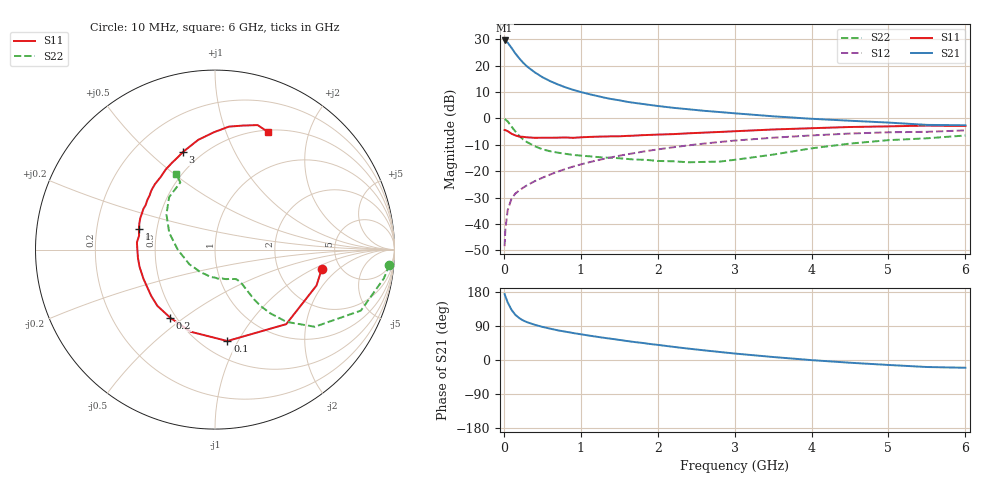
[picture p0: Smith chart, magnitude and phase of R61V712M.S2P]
! SIEMENS Small Signal Semiconductors
! BFR193
! Si NPN RF Bipolar Junction Transistor in SOT23
! VCE = 1.75 V  IC = 12 mA
! Common Emitter S-Parameters:  May  1996
# GHz  S  MA  R  50
!  f  S11  S21  S12  S22
! GHz  MAG  ANG  MAG  ANG  MAG  ANG  MAG  ANG
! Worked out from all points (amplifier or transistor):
!   36 points, 10 MHz to 6 GHz, reference 50 ohm
!   highest |S21| = 29.6 dB at 10 MHz (marker M1)
!   |S21| within 3 dB of that: start of sweep to 104.4 MHz
!   unconditionally stable (mu >= 1): 656.6 MHz to 1.947 GHz
!   at 250 MHz: K = 0.70, MSG = 23.7 dB, |S12| = -26.2 dB
!   at 1.4 GHz: K = 1.04, MAG = 9.9 dB, |S12| = -14.7 dB
!   at 6 GHz: K = 0.95, MSG = 1.0 dB, |S12| = -4.5 dB
!   S11 on the Smith chart (normalised r, x): 10 MHz: 3.62, -1.22; 100 MHz: 0.65, -0.90; 200 MHz: 0.47, -0.45; 1 GHz: 0.40, +0.11; 3 GHz: 0.40, +0.65; 6 GHz: 0.52, +1.41
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0.01  0.6046 -10.2  30.11 174.1  0.0038 87.0  0.9753 -4.9
0.02  0.5999 -19.5  29.45 168.1  0.0079 82.5  0.9544 -9.7
0.05  0.5744 -46.3  27.36 152.1  0.0184 71.9  0.8808 -22.7
0.1  0.514 -82.3  21.78 132.3  0.0302 60.9  0.7029 -37.7
0.15  0.4773 -106.5  17.02 119.1  0.0379 57.2  0.5665 -45.3
0.2  0.4541 -123.3  13.83 110.6  0.0432 56.4  0.469 -49.1
0.25  0.4488 -135.7  11.43 104.4  0.0487 56.7  0.4012 -51.1
0.3  0.439 -144.2  9.731 99.9  0.054 57.7  0.3576 -51.8
0.4  0.4305 -157.7  7.53 93.1  0.0646 59.9  0.2987 -51.9
0.5  0.4313 -167.2  6.083 87.5  0.0752 61.7  0.2607 -51.8
0.6  0.4318 -173.8  5.12 82.8  0.0864 62.9  0.2394 -51.9
0.7  0.4332 179.1  4.437 78.4  0.098 63.7  0.2253 -52.4
0.8  0.4369 174.6  3.896 74.8  0.1102 63.7  0.2139 -53.3
1  0.4392 165.0  3.174 67.9  0.1346 63.7  0.1977 -55.9
1.1  0.4462 160.8  2.916 64.7  0.1468 63.2  0.1925 -58.4
1.6  0.4675 143.8  2.073 50.1  0.2088 59.3  0.1713 -72.4
2.2  0.505 126.9  1.595 34.8  0.2844 52.4  0.1544 -98.7
3  0.5725 108.2  1.254 17.1  0.381 41.0  0.1644 -149.8
3.5  0.6186 98.7  1.1 7.9  0.4319 33.2  0.2068 -179.6
4.5  0.6894 83.6  0.906 -7.2  0.5179 18.4  0.3343 144.0
5.5  0.7333 71.1  0.756 -18.5  0.5587 3.5  0.4212 117.3
6  0.7192 66.0  0.743 -20.5  0.5945 -0.9  0.476 117.2
